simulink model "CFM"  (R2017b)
settings: Solver=FixedStepDiscrete  StartTime=0.0  StopTime=10.0  FixedStep=0.01  RelTol=1e-3  EnableMultiTasking=on
undefined symbols (not defined in the file): ASWTYPE_FALSE, CaCFM_BusBarCell_enum, CaCFM_NTCTemp_enum, CcCFM_AFEAdcRelatedErrDeb_ms, CcCFM_AFECellTempUpdErrDeb_ms, CcCFM_AFECellVoltLineOpenDeb_ms, CcCFM_AFECellVoltUpdErrDeb_ms, CcCFM_AFEComLostDeb_ms, CcCFM_AFEDiagModeExitErrDeb_ms, CcCFM_AFEGpioLineOpenDeb_ms, CcCFM_AFEOtherErrDeb_ms, CcCFM_AFESampleErrDeb_ms, CFM_CONST0_NUMB, CFM_CONST14_NUMB, CFM_CONST1_NUMB, CFM_CONST6_NUMB, CFM_CONST8_NUMB, CFM_RUNTIME20_MS, Enum_CFMBusBarCell, Enum_CFMNTCTemp
libraries: AIWAYS_Powertrain_BMS_lib x22

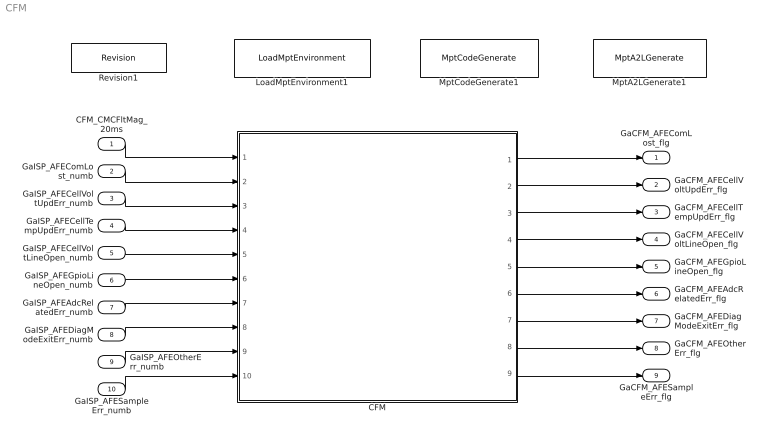
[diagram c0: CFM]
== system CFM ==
  CFM_CMCFltMag_20ms : Inport
  GaISP_AFEComLost_numb : Inport  Port=2
  GaISP_AFECellVoltUpdErr_numb : Inport  Port=3
  GaISP_AFECellTempUpdErr_numb : Inport  Port=4
  GaISP_AFECellVoltLineOpen_numb : Inport  Port=5
  GaISP_AFEGpioLineOpen_numb : Inport  Port=6
  GaISP_AFEAdcRelatedErr_numb : Inport  Port=7
  GaISP_AFEDiagModeExitErr_numb : Inport  Port=8
  GaISP_AFEOtherErr_numb : Inport  Port=9
  GaISP_AFESampleErr_numb : Inport  Port=10
  CFM : Subsystem
  LoadMptEnvironment1 : AIWAYS_Powertrain_BMS_lib/Config/LoadMptEnvironment  ProjectName=861B  SuppierID=NewPlatformUAES
  MptA2LGenerate1 : AIWAYS_Powertrain_BMS_lib/Config/MptA2LGenerate  SystemSampleTime=-1
  MptCodeGenerate1 : AIWAYS_Powertrain_BMS_lib/Config/MptCodeGenerate  SystemSampleTime=-1
  Revision1 : AIWAYS_Powertrain_BMS_lib/Config/Revision  curVersion='M100C100'  newVersion='M100C100'
  GaCFM_AFEComLost_flg : Outport
  GaCFM_AFECellVoltUpdErr_flg : Outport  Port=2
  GaCFM_AFECellTempUpdErr_flg : Outport  Port=3
  GaCFM_AFECellVoltLineOpen_flg : Outport  Port=4
  GaCFM_AFEGpioLineOpen_flg : Outport  Port=5
  GaCFM_AFEAdcRelatedErr_flg : Outport  Port=6
  GaCFM_AFEDiagModeExitErr_flg : Outport  Port=7
  GaCFM_AFEOtherErr_flg : Outport  Port=8
  GaCFM_AFESampleErr_flg : Outport  Port=9
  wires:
  GaISP_AFEComLost_numb/1 -> CFM/2(GaISP_AFEComLost_numb)
  GaISP_AFECellVoltUpdErr_numb/1 -> CFM/3(GaISP_AFECellVoltUpdErr_numb)
  GaISP_AFECellTempUpdErr_numb/1 -> CFM/4(GaISP_AFECellTempUpdErr_numb)
  GaISP_AFECellVoltLineOpen_numb/1 -> CFM/5(GaISP_AFECellVoltLineOpen_numb)
  GaISP_AFEGpioLineOpen_numb/1 -> CFM/6(GaISP_AFEGpioLineOpen_numb)
  GaISP_AFEAdcRelatedErr_numb/1 -> CFM/7(GaISP_AFEAdcRelatedErr_numb)
  GaISP_AFEDiagModeExitErr_numb/1 -> CFM/8(GaISP_AFEDiagModeExitErr_numb)
  GaISP_AFEOtherErr_numb/1 -> CFM/9(GaISP_AFEOtherErr_numb)
  GaISP_AFESampleErr_numb/1 -> CFM/10(GaISP_AFESampleErr_numb)
  CFM_CMCFltMag_20ms/1 -> CFM/1(CFM_CMCFltMag_20ms)
  CFM/1(GaCFM_AFEComLost_flg) -> GaCFM_AFEComLost_flg/1
  CFM/2(GaCFM_AFECellVoltUpdErr_flg) -> GaCFM_AFECellVoltUpdErr_flg/1
  CFM/3(GaCFM_AFECellTempUpdErr_flg) -> GaCFM_AFECellTempUpdErr_flg/1
  CFM/4(GaCFM_AFECellVoltLineOpen_flg) -> GaCFM_AFECellVoltLineOpen_flg/1
  CFM/5(GaCFM_AFEGpioLineOpen_flg) -> GaCFM_AFEGpioLineOpen_flg/1
  CFM/6(GaCFM_AFEAdcRelatedErr_flg) -> GaCFM_AFEAdcRelatedErr_flg/1
  CFM/7(GaCFM_AFEDiagModeExitErr_flg) -> GaCFM_AFEDiagModeExitErr_flg/1
  CFM/8(GaCFM_AFEOtherErr_flg) -> GaCFM_AFEOtherErr_flg/1
  CFM/9(GaCFM_AFESampleErr_flg) -> GaCFM_AFESampleErr_flg/1

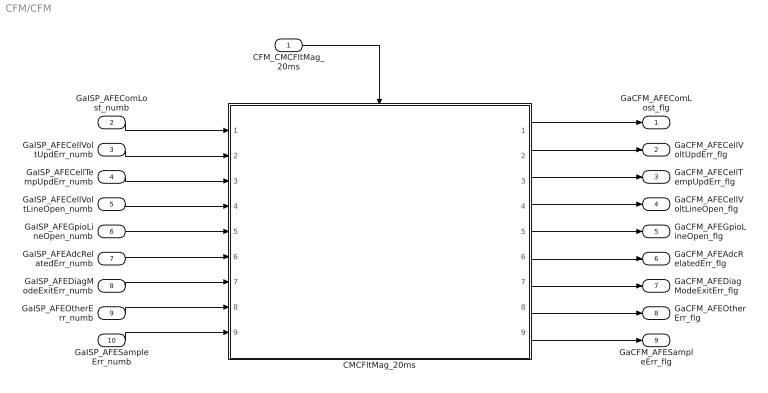
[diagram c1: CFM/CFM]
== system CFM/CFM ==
  CFM_CMCFltMag_20ms : Inport
  GaISP_AFEComLost_numb : Inport  Port=2
  GaISP_AFECellVoltUpdErr_numb : Inport  Port=3
  GaISP_AFECellTempUpdErr_numb : Inport  Port=4
  GaISP_AFECellVoltLineOpen_numb : Inport  Port=5
  GaISP_AFEGpioLineOpen_numb : Inport  Port=6
  GaISP_AFEAdcRelatedErr_numb : Inport  Port=7
  GaISP_AFEDiagModeExitErr_numb : Inport  Port=8
  GaISP_AFEOtherErr_numb : Inport  Port=9
  GaISP_AFESampleErr_numb : Inport  Port=10
  CMCFltMag_20ms : Subsystem
  GaCFM_AFEComLost_flg : Outport
  GaCFM_AFECellVoltUpdErr_flg : Outport  Port=2
  GaCFM_AFECellTempUpdErr_flg : Outport  Port=3
  GaCFM_AFECellVoltLineOpen_flg : Outport  Port=4
  GaCFM_AFEGpioLineOpen_flg : Outport  Port=5
  GaCFM_AFEAdcRelatedErr_flg : Outport  Port=6
  GaCFM_AFEDiagModeExitErr_flg : Outport  Port=7
  GaCFM_AFEOtherErr_flg : Outport  Port=8
  GaCFM_AFESampleErr_flg : Outport  Port=9
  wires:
  CFM_CMCFltMag_20ms/1 -> CMCFltMag_20ms/Trigger
  GaISP_AFEComLost_numb/1 -> CMCFltMag_20ms/1(GaISP_AFEComLost_numb)
  GaISP_AFECellVoltUpdErr_numb/1 -> CMCFltMag_20ms/2(GaISP_AFECellVoltUpdErr_numb)
  GaISP_AFECellTempUpdErr_numb/1 -> CMCFltMag_20ms/3(GaISP_AFECellTempUpdErr_numb)
  GaISP_AFECellVoltLineOpen_numb/1 -> CMCFltMag_20ms/4(GaISP_AFECellVoltLineOpen_numb)
  GaISP_AFEGpioLineOpen_numb/1 -> CMCFltMag_20ms/5(GaISP_AFEGpioLineOpen_numb)
  GaISP_AFEAdcRelatedErr_numb/1 -> CMCFltMag_20ms/6(GaISP_AFEAdcRelatedErr_numb)
  GaISP_AFEDiagModeExitErr_numb/1 -> CMCFltMag_20ms/7(GaISP_AFEDiagModeExitErr_numb)
  GaISP_AFEOtherErr_numb/1 -> CMCFltMag_20ms/8(GaISP_AFEOtherErr_numb)
  GaISP_AFESampleErr_numb/1 -> CMCFltMag_20ms/9(GaISP_AFESampleErr_numb)
  CMCFltMag_20ms/1(GaCFM_AFEComLost_flg) -> GaCFM_AFEComLost_flg/1
  CMCFltMag_20ms/2(GaCFM_AFECellVoltUpdErr_flg) -> GaCFM_AFECellVoltUpdErr_flg/1
  CMCFltMag_20ms/3(GaCFM_AFECellTempUpdErr_flg) -> GaCFM_AFECellTempUpdErr_flg/1
  CMCFltMag_20ms/4(GaCFM_AFECellVoltLineOpen_flg) -> GaCFM_AFECellVoltLineOpen_flg/1
  CMCFltMag_20ms/5(GaCFM_AFEGpioLineOpen_flg) -> GaCFM_AFEGpioLineOpen_flg/1
  CMCFltMag_20ms/6(GaCFM_AFEAdcRelatedErr_flg) -> GaCFM_AFEAdcRelatedErr_flg/1
  CMCFltMag_20ms/7(GaCFM_AFEDiagModeExitErr_flg) -> GaCFM_AFEDiagModeExitErr_flg/1
  CMCFltMag_20ms/8(GaCFM_AFEOtherErr_flg) -> GaCFM_AFEOtherErr_flg/1
  CMCFltMag_20ms/9(GaCFM_AFESampleErr_flg) -> GaCFM_AFESampleErr_flg/1

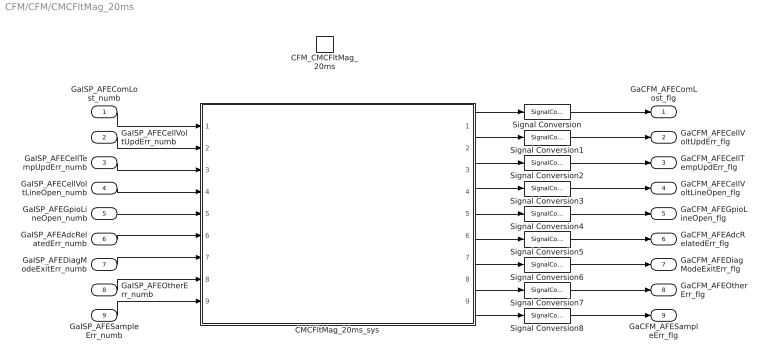
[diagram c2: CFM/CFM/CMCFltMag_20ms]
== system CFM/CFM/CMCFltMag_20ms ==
  GaISP_AFEComLost_numb : Inport
  GaISP_AFECellVoltUpdErr_numb : Inport  Port=2
  GaISP_AFECellTempUpdErr_numb : Inport  Port=3
  GaISP_AFECellVoltLineOpen_numb : Inport  Port=4
  GaISP_AFEGpioLineOpen_numb : Inport  Port=5
  GaISP_AFEAdcRelatedErr_numb : Inport  Port=6
  GaISP_AFEDiagModeExitErr_numb : Inport  Port=7
  GaISP_AFEOtherErr_numb : Inport  Port=8
  GaISP_AFESampleErr_numb : Inport  Port=9
  CFM_CMCFltMag_20ms : TriggerPort  TriggerType=function-call  VariantControl=(inherit)
  CMCFltMag_20ms_sys : Subsystem
  Signal Conversion{,1..8} (9 alike) : SignalConversion  ConversionOutput=Contiguous copy  OverrideOpt=off
  GaCFM_AFEComLost_flg : Outport
  GaCFM_AFECellVoltUpdErr_flg : Outport  Port=2
  GaCFM_AFECellTempUpdErr_flg : Outport  Port=3
  GaCFM_AFECellVoltLineOpen_flg : Outport  Port=4
  GaCFM_AFEGpioLineOpen_flg : Outport  Port=5
  GaCFM_AFEAdcRelatedErr_flg : Outport  Port=6
  GaCFM_AFEDiagModeExitErr_flg : Outport  Port=7
  GaCFM_AFEOtherErr_flg : Outport  Port=8
  GaCFM_AFESampleErr_flg : Outport  Port=9
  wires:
  GaISP_AFEComLost_numb/1 -> CMCFltMag_20ms_sys/1(GaISP_AFEComLost_numb)
  GaISP_AFECellVoltUpdErr_numb/1 -> CMCFltMag_20ms_sys/2(GaISP_AFECellVoltUpdErr_numb)
  GaISP_AFECellTempUpdErr_numb/1 -> CMCFltMag_20ms_sys/3(GaISP_AFECellTempUpdErr_numb)
  GaISP_AFECellVoltLineOpen_numb/1 -> CMCFltMag_20ms_sys/4(GaISP_AFECellVoltLineOpen_numb)
  GaISP_AFEGpioLineOpen_numb/1 -> CMCFltMag_20ms_sys/5(GaISP_AFEGpioLineOpen_numb)
  GaISP_AFEAdcRelatedErr_numb/1 -> CMCFltMag_20ms_sys/6(GaISP_AFEAdcRelatedErr_numb)
  GaISP_AFEDiagModeExitErr_numb/1 -> CMCFltMag_20ms_sys/7(GaISP_AFEDiagModeExitErr_numb)
  GaISP_AFEOtherErr_numb/1 -> CMCFltMag_20ms_sys/8(GaISP_AFEOtherErr_numb)
  GaISP_AFESampleErr_numb/1 -> CMCFltMag_20ms_sys/9(GaISP_AFESampleErr_numb)
  CMCFltMag_20ms_sys/1(GaCFM_AFEComLost_flg) -> Signal Conversion/1
  CMCFltMag_20ms_sys/2(GaCFM_AFECellVoltUpdErr_flg) -> Signal Conversion1/1
  CMCFltMag_20ms_sys/3(GaCFM_AFECellTempUpdErr_flg) -> Signal Conversion2/1
  CMCFltMag_20ms_sys/4(GaCFM_AFECellVoltLineOpen_flg) -> Signal Conversion3/1
  CMCFltMag_20ms_sys/5(GaCFM_AFEGpioLineOpen_flg) -> Signal Conversion4/1
  CMCFltMag_20ms_sys/6(GaCFM_AFEAdcRelatedErr_flg) -> Signal Conversion5/1
  CMCFltMag_20ms_sys/7(GaCFM_AFEDiagModeExitErr_flg) -> Signal Conversion6/1
  CMCFltMag_20ms_sys/8(GaCFM_AFEOtherErr_flg) -> Signal Conversion7/1
  CMCFltMag_20ms_sys/9(GaCFM_AFESampleErr_flg) -> Signal Conversion8/1
  Signal Conversion/1 -> GaCFM_AFEComLost_flg/1
  Signal Conversion1/1 -> GaCFM_AFECellVoltUpdErr_flg/1
  Signal Conversion2/1 -> GaCFM_AFECellTempUpdErr_flg/1
  Signal Conversion3/1 -> GaCFM_AFECellVoltLineOpen_flg/1
  Signal Conversion4/1 -> GaCFM_AFEGpioLineOpen_flg/1
  Signal Conversion5/1 -> GaCFM_AFEAdcRelatedErr_flg/1
  Signal Conversion6/1 -> GaCFM_AFEDiagModeExitErr_flg/1
  Signal Conversion7/1 -> GaCFM_AFEOtherErr_flg/1
  Signal Conversion8/1 -> GaCFM_AFESampleErr_flg/1

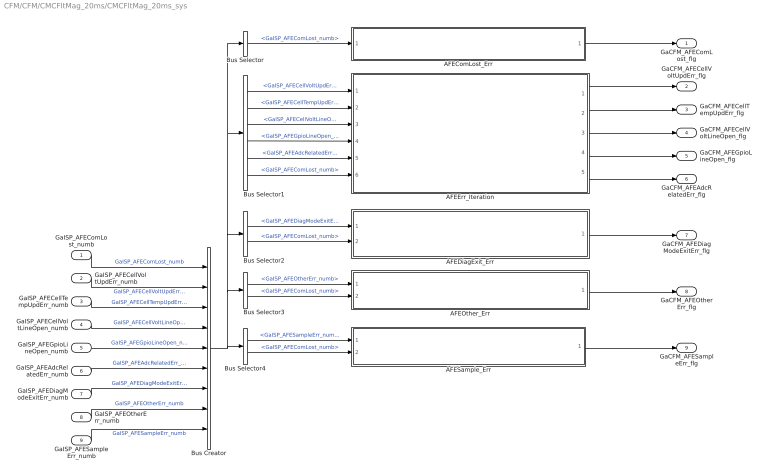
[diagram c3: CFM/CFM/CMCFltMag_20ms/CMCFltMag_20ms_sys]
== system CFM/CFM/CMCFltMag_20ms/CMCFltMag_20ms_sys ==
  GaISP_AFEComLost_numb : Inport
  GaISP_AFECellVoltUpdErr_numb : Inport  Port=2
  GaISP_AFECellTempUpdErr_numb : Inport  Port=3
  GaISP_AFECellVoltLineOpen_numb : Inport  Port=4
  GaISP_AFEGpioLineOpen_numb : Inport  Port=5
  GaISP_AFEAdcRelatedErr_numb : Inport  Port=6
  GaISP_AFEDiagModeExitErr_numb : Inport  Port=7
  GaISP_AFEOtherErr_numb : Inport  Port=8
  GaISP_AFESampleErr_numb : Inport  Port=9
  AFEComLost_Err : Subsystem
  AFEDiagExit_Err : Subsystem
  AFEErr_Iteration : Subsystem
  AFEOther_Err : Subsystem
  AFESample_Err : Subsystem
  Bus Creator : BusCreator  Inputs=9
  Bus Selector : BusSelector  OutputSignals=GaISP_AFEComLost_numb
  Bus Selector1 : BusSelector  OutputSignals=GaISP_AFECellVoltUpdErr_numb,GaISP_AFECellTempUpdErr_numb,GaISP_AFECellVoltLineOpen_numb,GaISP_AFEGpioLineOpen_numb,GaISP_AFEAdcRelatedErr_numb,GaISP_AFEComLost_numb
  Bus Selector2 : BusSelector  OutputSignals=GaISP_AFEDiagModeExitErr_numb,GaISP_AFEComLost_numb
  Bus Selector3 : BusSelector  OutputSignals=GaISP_AFEOtherErr_numb,GaISP_AFEComLost_numb
  Bus Selector4 : BusSelector  OutputSignals=GaISP_AFESampleErr_numb,GaISP_AFEComLost_numb
  GaCFM_AFEComLost_flg : Outport
  GaCFM_AFECellVoltUpdErr_flg : Outport  Port=2
  GaCFM_AFECellTempUpdErr_flg : Outport  Port=3
  GaCFM_AFECellVoltLineOpen_flg : Outport  Port=4
  GaCFM_AFEGpioLineOpen_flg : Outport  Port=5
  GaCFM_AFEAdcRelatedErr_flg : Outport  Port=6
  GaCFM_AFEDiagModeExitErr_flg : Outport  Port=7
  GaCFM_AFEOtherErr_flg : Outport  Port=8
  GaCFM_AFESampleErr_flg : Outport  Port=9
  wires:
  AFEComLost_Err/1(GaCFM_AFEComLost_flg) -> GaCFM_AFEComLost_flg/1
  AFEDiagExit_Err/1(GaCFM_AFEDiagModeExitErr_flg) -> GaCFM_AFEDiagModeExitErr_flg/1
  AFEOther_Err/1(GaCFM_AFEOtherErr_flg) -> GaCFM_AFEOtherErr_flg/1
  AFESample_Err/1(GaCFM_AFESampleErr_flg) -> GaCFM_AFESampleErr_flg/1
  AFEErr_Iteration/1(GaCFM_AFECellVoltUpdErr_flg) -> GaCFM_AFECellVoltUpdErr_flg/1
  AFEErr_Iteration/2(GaCFM_AFECellTempUpdErr_flg) -> GaCFM_AFECellTempUpdErr_flg/1
  AFEErr_Iteration/3(GaCFM_AFECellVoltLineOpen_flg) -> GaCFM_AFECellVoltLineOpen_flg/1
  AFEErr_Iteration/4(GaCFM_AFEGpioLineOpen_flg) -> GaCFM_AFEGpioLineOpen_flg/1
  AFEErr_Iteration/5(GaCFM_AFEAdcRelatedErr_flg) -> GaCFM_AFEAdcRelatedErr_flg/1
  GaISP_AFEComLost_numb/1 -> Bus Creator/1  "GaISP_AFEComLost_numb"
  GaISP_AFECellVoltUpdErr_numb/1 -> Bus Creator/2  "GaISP_AFECellVoltUpdErr_numb"
  GaISP_AFECellTempUpdErr_numb/1 -> Bus Creator/3  "GaISP_AFECellTempUpdErr_numb"
  GaISP_AFECellVoltLineOpen_numb/1 -> Bus Creator/4  "GaISP_AFECellVoltLineOpen_numb"
  GaISP_AFEGpioLineOpen_numb/1 -> Bus Creator/5  "GaISP_AFEGpioLineOpen_numb"
  GaISP_AFEAdcRelatedErr_numb/1 -> Bus Creator/6  "GaISP_AFEAdcRelatedErr_numb"
  GaISP_AFEDiagModeExitErr_numb/1 -> Bus Creator/7  "GaISP_AFEDiagModeExitErr_numb"
  GaISP_AFEOtherErr_numb/1 -> Bus Creator/8  "GaISP_AFEOtherErr_numb"
  GaISP_AFESampleErr_numb/1 -> Bus Creator/9  "GaISP_AFESampleErr_numb"
  Bus Creator/1 -> Bus Selector/1, Bus Selector1/1, Bus Selector2/1, Bus Selector3/1, Bus Selector4/1
  Bus Selector/1 -> AFEComLost_Err/1(GaISP_AFEComLost_numb)  "<GaISP_AFEComLost_numb>"
  Bus Selector1/1 -> AFEErr_Iteration/1(GaISP_AFECellVoltUpdErr_numb)  "<GaISP_AFECellVoltUpdErr_numb>"
  Bus Selector1/2 -> AFEErr_Iteration/2(GaISP_AFECellTempUpdErr_numb)  "<GaISP_AFECellTempUpdErr_numb>"
  Bus Selector1/3 -> AFEErr_Iteration/3(GaISP_AFECellVoltLineOpen_numb)  "<GaISP_AFECellVoltLineOpen_numb>"
  Bus Selector1/4 -> AFEErr_Iteration/4(GaISP_AFEGpioLineOpen_numb)  "<GaISP_AFEGpioLineOpen_numb>"
  Bus Selector1/5 -> AFEErr_Iteration/5(GaISP_AFEAdcRelatedErr_numb)  "<GaISP_AFEAdcRelatedErr_numb>"
  Bus Selector1/6 -> AFEErr_Iteration/6(GaISP_AFEComLost_numb)  "<GaISP_AFEComLost_numb>"
  Bus Selector2/1 -> AFEDiagExit_Err/1(GaISP_AFEDiagModeExitErr_numb)  "<GaISP_AFEDiagModeExitErr_numb>"
  Bus Selector2/2 -> AFEDiagExit_Err/2(GaISP_AFEComLost_numb)  "<GaISP_AFEComLost_numb>"
  Bus Selector3/1 -> AFEOther_Err/1(GaISP_AFEOtherErr_numb)  "<GaISP_AFEOtherErr_numb>"
  Bus Selector3/2 -> AFEOther_Err/2(GaISP_AFEComLost_numb)  "<GaISP_AFEComLost_numb>"
  Bus Selector4/2 -> AFESample_Err/2(GaISP_AFEComLost_numb)  "<GaISP_AFEComLost_numb>"
  Bus Selector4/1 -> AFESample_Err/1(GaISP_AFESampleErr_numb)  "<GaISP_AFESampleErr_numb>"

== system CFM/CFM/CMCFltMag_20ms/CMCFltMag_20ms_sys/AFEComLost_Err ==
  GaISP_AFEComLost_numb : Inport
  BMSDelay : AIWAYS_Powertrain_BMS_lib/Debounce & Delay/BMSDelay
  CFM_GaCFM_AFEComLost_flg : AIWAYS_Powertrain_BMS_lib/Signals/OverWrite  OverWrite_Value=CaCFM_AFEComLostOvr_flg  OverWrite_flag=CbCFM_AFEComLostOvrSwt_flg
  Constant1 : Constant  Value=CFM_RUNTIME20_MS
  Constant3 : Constant  Value=CFM_CONST0_NUMB
  Constant5 : Constant  Value=CcCFM_AFEComLostDeb_ms
  Relational Operator2 : RelationalOperator  Operator=~=  OutDataTypeStr=boolean
  GaCFM_AFEComLost_flg : Outport
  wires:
  GaISP_AFEComLost_numb/1 -> Relational Operator2/1
  Constant3/1 -> Relational Operator2/2
  CFM_GaCFM_AFEComLost_flg/1 -> GaCFM_AFEComLost_flg/1  "GaCFM_AFEComLost_flg"
  Relational Operator2/1 -> BMSDelay/1  "LaCFM_AFEComLost_flg"
  BMSDelay/1 -> CFM_GaCFM_AFEComLost_flg/1
  Constant1/1 -> BMSDelay/2
  Constant5/1 -> BMSDelay/3

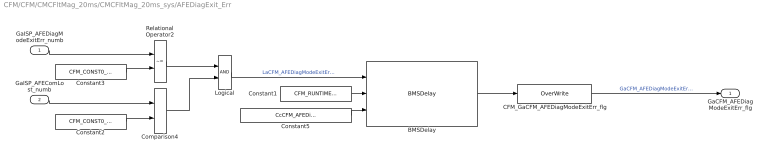
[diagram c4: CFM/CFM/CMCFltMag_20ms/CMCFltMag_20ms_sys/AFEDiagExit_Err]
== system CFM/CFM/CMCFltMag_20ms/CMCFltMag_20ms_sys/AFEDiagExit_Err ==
  GaISP_AFEDiagModeExitErr_numb : Inport
  GaISP_AFEComLost_numb : Inport  Port=2
  BMSDelay : AIWAYS_Powertrain_BMS_lib/Debounce & Delay/BMSDelay
  CFM_GaCFM_AFEDiagModeExitErr_flg : AIWAYS_Powertrain_BMS_lib/Signals/OverWrite  OverWrite_Value=CaCFM_AFEDiagModeExitErrOvr_flg  OverWrite_flag=CbCFM_AFEDiagModeExitErrOvrSwt_flg
  Comparison4 : RelationalOperator  Operator===  OutDataTypeStr=boolean
  Constant1 : Constant  Value=CFM_RUNTIME20_MS
  Constant2 : Constant  Value=CFM_CONST0_NUMB
  Constant3 : Constant  Value=CFM_CONST0_NUMB
  Constant5 : Constant  Value=CcCFM_AFEDiagModeExitErrDeb_ms
  Logical : Logic  OutDataTypeStr=boolean
  Relational Operator2 : RelationalOperator  Operator=~=  OutDataTypeStr=boolean
  GaCFM_AFEDiagModeExitErr_flg : Outport
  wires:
  Constant3/1 -> Relational Operator2/2
  GaISP_AFEDiagModeExitErr_numb/1 -> Relational Operator2/1
  CFM_GaCFM_AFEDiagModeExitErr_flg/1 -> GaCFM_AFEDiagModeExitErr_flg/1  "GaCFM_AFEDiagModeExitErr_flg"
  Constant5/1 -> BMSDelay/3
  Constant1/1 -> BMSDelay/2
  BMSDelay/1 -> CFM_GaCFM_AFEDiagModeExitErr_flg/1
  Constant2/1 -> Comparison4/2
  GaISP_AFEComLost_numb/1 -> Comparison4/1
  Relational Operator2/1 -> Logical/1
  Comparison4/1 -> Logical/2
  Logical/1 -> BMSDelay/1  "LaCFM_AFEDiagModeExitErr_flg"

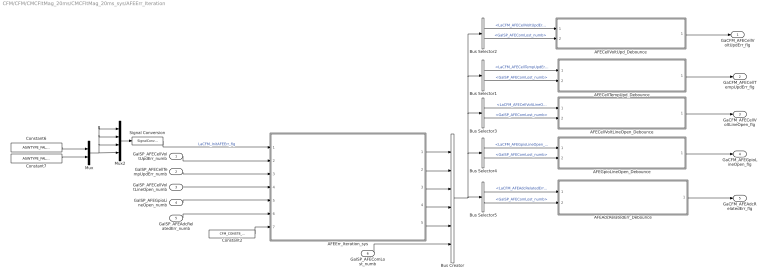
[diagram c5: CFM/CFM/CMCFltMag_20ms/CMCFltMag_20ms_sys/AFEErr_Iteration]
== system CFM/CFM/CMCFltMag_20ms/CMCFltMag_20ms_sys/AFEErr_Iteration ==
  GaISP_AFECellVoltUpdErr_numb : Inport
  GaISP_AFECellTempUpdErr_numb : Inport  Port=2
  GaISP_AFECellVoltLineOpen_numb : Inport  Port=3
  GaISP_AFEGpioLineOpen_numb : Inport  Port=4
  GaISP_AFEAdcRelatedErr_numb : Inport  Port=5
  GaISP_AFEComLost_numb : Inport  Port=6
  AFEAdcRelatedErr_Debounce : Subsystem
  AFECellTempUpd_Debounce : Subsystem
  AFECellVoltLineOpen_Debounce : Subsystem
  AFECellVoltUpd_Debounce : Subsystem
  AFEErr_Iteration_sys : Subsystem
  AFEGpioLineOpen_Debounce : Subsystem
  Bus Creator : BusCreator  Inputs=6
  Bus Selector1 : BusSelector  OutputSignals=LaCFM_AFECellTempUpdErr_flg,GaISP_AFEComLost_numb
  Bus Selector2 : BusSelector  OutputSignals=LaCFM_AFECellVoltUpdErr_flg,GaISP_AFEComLost_numb
  Bus Selector3 : BusSelector  OutputSignals=LaCFM_AFECellVoltLineOpen_flg,GaISP_AFEComLost_numb
  Bus Selector4 : BusSelector  OutputSignals=LaCFM_AFEGpioLineOpen_flg,GaISP_AFEComLost_numb
  Bus Selector5 : BusSelector  OutputSignals=LaCFM_AFEAdcRelatedErr_flg,GaISP_AFEComLost_numb
  Constant2 : Constant  Value=CFM_CONST8_NUMB
  Constant6 : Constant  Value=ASWTYPE_FALSE
  Constant7 : Constant  Value=ASWTYPE_FALSE
  Mux : Mux  Inputs=2
  Mux2 : Mux
  Signal Conversion : SignalConversion  ConversionOutput=Contiguous copy  OverrideOpt=off
  GaCFM_AFECellVoltUpdErr_flg : Outport
  GaCFM_AFECellTempUpdErr_flg : Outport  Port=2
  GaCFM_AFECellVoltLineOpen_flg : Outport  Port=3
  GaCFM_AFEGpioLineOpen_flg : Outport  Port=4
  GaCFM_AFEAdcRelatedErr_flg : Outport  Port=5
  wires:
  GaISP_AFEGpioLineOpen_numb/1 -> AFEErr_Iteration_sys/5(GaISP_AFEGpioLineOpen_numb)
  GaISP_AFECellTempUpdErr_numb/1 -> AFEErr_Iteration_sys/3(GaISP_AFECellTempUpdErr_numb)
  Signal Conversion/1 -> AFEErr_Iteration_sys/1(LaCFM_InitAFEErr_flg)  "LaCFM_InitAFEErr_flg"
  GaISP_AFECellVoltLineOpen_numb/1 -> AFEErr_Iteration_sys/4(GaISP_AFECellVoltLineOpen_numb)
  Constant2/1 -> AFEErr_Iteration_sys/7(CFM_CONST8_NUMB)
  GaISP_AFECellVoltUpdErr_numb/1 -> AFEErr_Iteration_sys/2(GaISP_AFECellVoltUpdErr_numb)
  GaISP_AFEAdcRelatedErr_numb/1 -> AFEErr_Iteration_sys/6(GaISP_AFEAdcRelatedErr_numb)
  Constant6/1 -> Mux/1
  Mux2/1 -> Signal Conversion/1
  Mux/1 -> Mux2/1, Mux2/2, Mux2/3, Mux2/4
  Constant7/1 -> Mux/2
  AFECellVoltUpd_Debounce/1(GaCFM_AFECellVoltUpdErr_flg) -> GaCFM_AFECellVoltUpdErr_flg/1
  AFECellTempUpd_Debounce/1(GaCFM_AFECellTempUpdErr_flg) -> GaCFM_AFECellTempUpdErr_flg/1
  AFECellVoltLineOpen_Debounce/1(GaCFM_AFECellVoltLineOpen_flg) -> GaCFM_AFECellVoltLineOpen_flg/1
  AFEGpioLineOpen_Debounce/1(GaCFM_AFEGpioLineOpen_flg) -> GaCFM_AFEGpioLineOpen_flg/1
  AFEAdcRelatedErr_Debounce/1(GaCFM_AFEAdcRelatedErr_flg) -> GaCFM_AFEAdcRelatedErr_flg/1
  AFEErr_Iteration_sys/1(LaCFM_AFECellVoltUpdErr_flg) -> Bus Creator/1
  AFEErr_Iteration_sys/2(LaCFM_AFECellTempUpdErr_flg) -> Bus Creator/2
  AFEErr_Iteration_sys/3(LaCFM_AFECellVoltLineOpen_flg) -> Bus Creator/3
  AFEErr_Iteration_sys/4(LaCFM_AFEGpioLineOpen_flg) -> Bus Creator/4
  AFEErr_Iteration_sys/5(LaCFM_AFEAdcRelatedErr_flg) -> Bus Creator/5
  GaISP_AFEComLost_numb/1 -> Bus Creator/6
  Bus Creator/1 -> Bus Selector1/1, Bus Selector2/1, Bus Selector3/1, Bus Selector4/1, Bus Selector5/1
  Bus Selector2/1 -> AFECellVoltUpd_Debounce/1(LaCFM_AFECellVoltUpdErr_flg)  "<LaCFM_AFECellVoltUpdErr_flg>"
  Bus Selector2/2 -> AFECellVoltUpd_Debounce/2(GaISP_AFEComLost_numb)  "<GaISP_AFEComLost_numb>"
  Bus Selector1/1 -> AFECellTempUpd_Debounce/1(LaCFM_AFECellTempUpdErr_flg)  "<LaCFM_AFECellTempUpdErr_flg>"
  Bus Selector1/2 -> AFECellTempUpd_Debounce/2(GaISP_AFEComLost_numb)  "<GaISP_AFEComLost_numb>"
  Bus Selector3/1 -> AFECellVoltLineOpen_Debounce/1(LaCFM_AFECellVoltLineOpen_flg)  "<LaCFM_AFECellVoltLineOpen_flg>"
  Bus Selector3/2 -> AFECellVoltLineOpen_Debounce/2(GaISP_AFEComLost_numb)  "<GaISP_AFEComLost_numb>"
  Bus Selector4/1 -> AFEGpioLineOpen_Debounce/1(LaCFM_AFEGpioLineOpen_flg)  "<LaCFM_AFEGpioLineOpen_flg>"
  Bus Selector4/2 -> AFEGpioLineOpen_Debounce/2(GaISP_AFEComLost_numb)  "<GaISP_AFEComLost_numb>"
  Bus Selector5/1 -> AFEAdcRelatedErr_Debounce/1(LaCFM_AFEAdcRelatedErr_flg)  "<LaCFM_AFEAdcRelatedErr_flg>"
  Bus Selector5/2 -> AFEAdcRelatedErr_Debounce/2(GaISP_AFEComLost_numb)  "<GaISP_AFEComLost_numb>"

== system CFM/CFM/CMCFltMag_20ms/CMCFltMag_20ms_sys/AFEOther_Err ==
  GaISP_AFEOtherErr_numb : Inport
  GaISP_AFEComLost_numb : Inport  Port=2
  BMSDelay : AIWAYS_Powertrain_BMS_lib/Debounce & Delay/BMSDelay
  CFM_GaCFM_AFEOtherErr_flg : AIWAYS_Powertrain_BMS_lib/Signals/OverWrite  OverWrite_Value=CaCFM_AFEOtherErrOvr_flg  OverWrite_flag=CbCFM_AFEOtherErrOvrSwt_flg
  Comparison4 : RelationalOperator  Operator===  OutDataTypeStr=boolean
  Constant1 : Constant  Value=CFM_RUNTIME20_MS
  Constant3 : Constant  Value=CFM_CONST0_NUMB
  Constant5 : Constant  Value=CcCFM_AFEOtherErrDeb_ms
  Constant6 : Constant  Value=CFM_CONST0_NUMB
  Logical : Logic  OutDataTypeStr=boolean
  Relational Operator2 : RelationalOperator  Operator=~=  OutDataTypeStr=boolean
  GaCFM_AFEOtherErr_flg : Outport
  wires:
  GaISP_AFEOtherErr_numb/1 -> Relational Operator2/1
  Constant3/1 -> Relational Operator2/2
  CFM_GaCFM_AFEOtherErr_flg/1 -> GaCFM_AFEOtherErr_flg/1  "GaCFM_AFEOtherErr_flg"
  Constant5/1 -> BMSDelay/3
  Constant1/1 -> BMSDelay/2
  BMSDelay/1 -> CFM_GaCFM_AFEOtherErr_flg/1
  Relational Operator2/1 -> Logical/1
  Constant6/1 -> Comparison4/2
  GaISP_AFEComLost_numb/1 -> Comparison4/1
  Comparison4/1 -> Logical/2
  Logical/1 -> BMSDelay/1  "LaCFM_AFEOtherErr_flg"

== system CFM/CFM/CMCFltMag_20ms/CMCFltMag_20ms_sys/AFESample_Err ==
  GaISP_AFESampleErr_numb : Inport
  GaISP_AFEComLost_numb : Inport  Port=2
  BMSDelay : AIWAYS_Powertrain_BMS_lib/Debounce & Delay/BMSDelay
  CFM_GaCFM_AFESampleErr_flg : AIWAYS_Powertrain_BMS_lib/Signals/OverWrite  OverWrite_Value=CaCFM_AFESampleErrOvr_flg  OverWrite_flag=CbCFM_AFESampleErrOvrSwt_flg
  Constant1 : Constant  Value=CFM_RUNTIME20_MS
  Constant2 : Constant  Value=CFM_CONST0_NUMB
  Constant3 : Constant  Value=CFM_CONST0_NUMB
  Constant5 : Constant  Value=CcCFM_AFESampleErrDeb_ms
  Logical : Logic  OutDataTypeStr=boolean
  Relational Operator1 : RelationalOperator  Operator===  OutDataTypeStr=boolean
  Relational Operator2 : RelationalOperator  Operator=~=  OutDataTypeStr=boolean
  GaCFM_AFESampleErr_flg : Outport
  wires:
  GaISP_AFESampleErr_numb/1 -> Relational Operator2/1
  Constant3/1 -> Relational Operator2/2
  CFM_GaCFM_AFESampleErr_flg/1 -> GaCFM_AFESampleErr_flg/1  "GaCFM_AFESampleErr_flg"
  Constant5/1 -> BMSDelay/3
  Constant1/1 -> BMSDelay/2
  BMSDelay/1 -> CFM_GaCFM_AFESampleErr_flg/1
  Logical/1 -> BMSDelay/1  "LaCFM_AFESampleErr_flg"
  Constant2/1 -> Relational Operator1/2
  GaISP_AFEComLost_numb/1 -> Relational Operator1/1
  Relational Operator2/1 -> Logical/1
  Relational Operator1/1 -> Logical/2

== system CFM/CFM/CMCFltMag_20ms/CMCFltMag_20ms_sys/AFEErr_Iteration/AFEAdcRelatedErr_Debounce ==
  LaCFM_AFEAdcRelatedErr_flg : Inport
  GaISP_AFEComLost_numb : Inport  Port=2
  BMSDelay : AIWAYS_Powertrain_BMS_lib/Debounce & Delay/BMSDelay
  CFM_GaCFM_AFEAdcRelatedErr_flg : AIWAYS_Powertrain_BMS_lib/Signals/OverWrite  OverWrite_Value=CaCFM_AFEAdcRelatedErrOvr_flg  OverWrite_flag=CbCFM_AFEAdcRelatedErrOvrSwt_flg
  Comparison4 : RelationalOperator  Operator===  OutDataTypeStr=boolean
  Constant1 : Constant  Value=CFM_RUNTIME20_MS
  Constant3 : Constant  Value=CFM_CONST0_NUMB
  Constant5 : Constant  Value=CcCFM_AFEAdcRelatedErrDeb_ms
  Logical : Logic  OutDataTypeStr=boolean
  GaCFM_AFEAdcRelatedErr_flg : Outport
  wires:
  LaCFM_AFEAdcRelatedErr_flg/1 -> Logical/1
  CFM_GaCFM_AFEAdcRelatedErr_flg/1 -> GaCFM_AFEAdcRelatedErr_flg/1  "GaCFM_AFEAdcRelatedErr_flg"
  BMSDelay/1 -> CFM_GaCFM_AFEAdcRelatedErr_flg/1
  Constant1/1 -> BMSDelay/2
  Constant5/1 -> BMSDelay/3
  GaISP_AFEComLost_numb/1 -> Comparison4/1
  Comparison4/1 -> Logical/2
  Logical/1 -> BMSDelay/1
  Constant3/1 -> Comparison4/2

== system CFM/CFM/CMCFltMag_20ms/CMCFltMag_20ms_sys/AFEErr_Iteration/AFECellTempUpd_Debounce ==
  LaCFM_AFECellTempUpdErr_flg : Inport
  GaISP_AFEComLost_numb : Inport  Port=2
  BMSDelay : AIWAYS_Powertrain_BMS_lib/Debounce & Delay/BMSDelay
  CFM_GaCFM_AFECellTempUpdErr_flg : AIWAYS_Powertrain_BMS_lib/Signals/OverWrite  OverWrite_Value=CaCFM_AFECellTempUpdErrOvr_flg  OverWrite_flag=CbCFM_AFECellTempUpdErrOvrSwt_flg
  Comparison4 : RelationalOperator  Operator===  OutDataTypeStr=boolean
  Constant1 : Constant  Value=CFM_RUNTIME20_MS
  Constant3 : Constant  Value=CFM_CONST0_NUMB
  Constant5 : Constant  Value=CcCFM_AFECellTempUpdErrDeb_ms
  Logical : Logic  OutDataTypeStr=boolean
  GaCFM_AFECellTempUpdErr_flg : Outport
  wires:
  CFM_GaCFM_AFECellTempUpdErr_flg/1 -> GaCFM_AFECellTempUpdErr_flg/1  "GaCFM_AFECellTempUpdErr_flg"
  BMSDelay/1 -> CFM_GaCFM_AFECellTempUpdErr_flg/1
  Constant5/1 -> BMSDelay/3
  Constant1/1 -> BMSDelay/2
  GaISP_AFEComLost_numb/1 -> Comparison4/1
  Comparison4/1 -> Logical/2
  LaCFM_AFECellTempUpdErr_flg/1 -> Logical/1
  Logical/1 -> BMSDelay/1
  Constant3/1 -> Comparison4/2

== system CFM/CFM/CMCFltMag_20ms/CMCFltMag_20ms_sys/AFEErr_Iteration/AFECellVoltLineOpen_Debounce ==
  LaCFM_AFECellVoltLineOpen_flg : Inport
  GaISP_AFEComLost_numb : Inport  Port=2
  BMSDelay : AIWAYS_Powertrain_BMS_lib/Debounce & Delay/BMSDelay
  CFM_GaCFM_AFECellVoltLineOpen_flg : AIWAYS_Powertrain_BMS_lib/Signals/OverWrite  OverWrite_Value=CaCFM_AFECellVoltLineOpenOvr_flg  OverWrite_flag=CbCFM_AFECellVoltLineOpenOvrSwt_flg
  Comparison4 : RelationalOperator  Operator===  OutDataTypeStr=boolean
  Constant1 : Constant  Value=CFM_RUNTIME20_MS
  Constant2 : Constant  Value=CFM_CONST0_NUMB
  Constant3 : Constant  Value=CcCFM_AFECellVoltLineOpenDeb_ms
  Logical : Logic  OutDataTypeStr=boolean
  GaCFM_AFECellVoltLineOpen_flg : Outport
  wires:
  LaCFM_AFECellVoltLineOpen_flg/1 -> Logical/1
  CFM_GaCFM_AFECellVoltLineOpen_flg/1 -> GaCFM_AFECellVoltLineOpen_flg/1  "GaCFM_AFECellVoltLineOpen_flg"
  BMSDelay/1 -> CFM_GaCFM_AFECellVoltLineOpen_flg/1
  Constant1/1 -> BMSDelay/2
  Constant3/1 -> BMSDelay/3
  GaISP_AFEComLost_numb/1 -> Comparison4/1
  Comparison4/1 -> Logical/2
  Logical/1 -> BMSDelay/1
  Constant2/1 -> Comparison4/2

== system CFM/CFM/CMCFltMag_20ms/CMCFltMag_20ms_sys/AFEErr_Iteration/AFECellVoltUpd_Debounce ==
  LaCFM_AFECellVoltUpdErr_flg : Inport
  GaISP_AFEComLost_numb : Inport  Port=2
  BMSDelay : AIWAYS_Powertrain_BMS_lib/Debounce & Delay/BMSDelay
  CFM_GaCFM_AFECellVoltUpdErr_flg : AIWAYS_Powertrain_BMS_lib/Signals/OverWrite  OverWrite_Value=CaCFM_AFECellVoltUpdErrOvr_flg  OverWrite_flag=CbCFM_AFECellVoltUpdErrOvrSwt_flg
  Comparison4 : RelationalOperator  Operator===  OutDataTypeStr=boolean
  Constant1 : Constant  Value=CFM_RUNTIME20_MS
  Constant3 : Constant  Value=CFM_CONST0_NUMB
  Constant5 : Constant  Value=CcCFM_AFECellVoltUpdErrDeb_ms
  Logical : Logic  OutDataTypeStr=boolean
  GaCFM_AFECellVoltUpdErr_flg : Outport
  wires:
  BMSDelay/1 -> CFM_GaCFM_AFECellVoltUpdErr_flg/1
  CFM_GaCFM_AFECellVoltUpdErr_flg/1 -> GaCFM_AFECellVoltUpdErr_flg/1  "GaCFM_AFECellVoltUpdErr_flg"
  Constant1/1 -> BMSDelay/2
  Constant5/1 -> BMSDelay/3
  Constant3/1 -> Comparison4/2
  GaISP_AFEComLost_numb/1 -> Comparison4/1
  Comparison4/1 -> Logical/2
  LaCFM_AFECellVoltUpdErr_flg/1 -> Logical/1
  Logical/1 -> BMSDelay/1

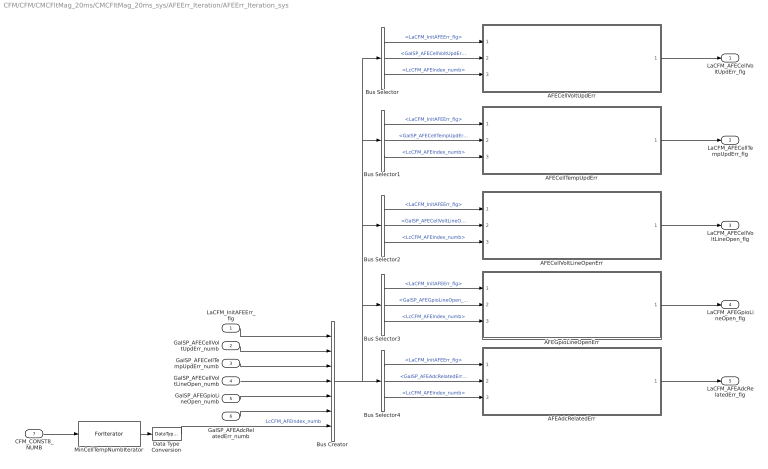
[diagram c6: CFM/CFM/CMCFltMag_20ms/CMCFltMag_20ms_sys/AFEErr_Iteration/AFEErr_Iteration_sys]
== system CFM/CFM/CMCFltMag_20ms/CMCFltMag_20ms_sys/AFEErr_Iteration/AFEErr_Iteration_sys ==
  LaCFM_InitAFEErr_flg : Inport
  GaISP_AFECellVoltUpdErr_numb : Inport  Port=2
  GaISP_AFECellTempUpdErr_numb : Inport  Port=3
  GaISP_AFECellVoltLineOpen_numb : Inport  Port=4
  GaISP_AFEGpioLineOpen_numb : Inport  Port=5
  GaISP_AFEAdcRelatedErr_numb : Inport  Port=6
  CFM_CONST8_NUMB : Inport  Port=7
  AFEAdcRelatedErr : Subsystem
  AFECellTempUpdErr : Subsystem
  AFECellVoltLineOpenErr : Subsystem
  AFECellVoltUpdErr : Subsystem
  AFEGpioLineOpenErr : Subsystem
  Bus Creator : BusCreator  Inputs=7
  Bus Selector : BusSelector  OutputSignals=LaCFM_InitAFEErr_flg,GaISP_AFECellVoltUpdErr_numb,LcCFM_AFEIndex_numb
  Bus Selector1 : BusSelector  OutputSignals=LaCFM_InitAFEErr_flg,GaISP_AFECellTempUpdErr_numb,LcCFM_AFEIndex_numb
  Bus Selector2 : BusSelector  OutputSignals=LaCFM_InitAFEErr_flg,GaISP_AFECellVoltLineOpen_numb,LcCFM_AFEIndex_numb
  Bus Selector3 : BusSelector  OutputSignals=LaCFM_InitAFEErr_flg,GaISP_AFEGpioLineOpen_numb,LcCFM_AFEIndex_numb
  Bus Selector4 : BusSelector  OutputSignals=LaCFM_InitAFEErr_flg,GaISP_AFEAdcRelatedErr_numb,LcCFM_AFEIndex_numb
  Data Type Conversion : DataTypeConversion  OutDataTypeStr=uint8
  MinCellTempNumbIterator : ForIterator  ResetStates=reset  IterationSource=external  IterationVariableDataType=int8
  LaCFM_AFECellVoltUpdErr_flg : Outport
  LaCFM_AFECellTempUpdErr_flg : Outport  Port=2
  LaCFM_AFECellVoltLineOpen_flg : Outport  Port=3
  LaCFM_AFEGpioLineOpen_flg : Outport  Port=4
  LaCFM_AFEAdcRelatedErr_flg : Outport  Port=5
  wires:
  MinCellTempNumbIterator/1 -> Data Type Conversion/1
  CFM_CONST8_NUMB/1 -> MinCellTempNumbIterator/1
  LaCFM_InitAFEErr_flg/1 -> Bus Creator/1
  GaISP_AFECellVoltUpdErr_numb/1 -> Bus Creator/2
  Data Type Conversion/1 -> Bus Creator/7  "LcCFM_AFEIndex_numb"
  Bus Creator/1 -> Bus Selector/1, Bus Selector1/1, Bus Selector2/1, Bus Selector3/1, Bus Selector4/1
  Bus Selector/1 -> AFECellVoltUpdErr/1(LaCFM_InitAFEErr_flg)  "<LaCFM_InitAFEErr_flg>"
  Bus Selector/2 -> AFECellVoltUpdErr/2(GaISP_AFECellVoltUpdErr_numb)  "<GaISP_AFECellVoltUpdErr_numb>"
  Bus Selector/3 -> AFECellVoltUpdErr/3(LcCFM_AFEIndex_numb)  "<LcCFM_AFEIndex_numb>"
  GaISP_AFECellTempUpdErr_numb/1 -> Bus Creator/3
  GaISP_AFECellVoltLineOpen_numb/1 -> Bus Creator/4
  GaISP_AFEGpioLineOpen_numb/1 -> Bus Creator/5
  GaISP_AFEAdcRelatedErr_numb/1 -> Bus Creator/6
  Bus Selector1/1 -> AFECellTempUpdErr/1(LaCFM_InitAFEErr_flg)  "<LaCFM_InitAFEErr_flg>"
  Bus Selector1/2 -> AFECellTempUpdErr/2(GaISP_AFECellTempUpdErr_numb)  "<GaISP_AFECellTempUpdErr_numb>"
  Bus Selector1/3 -> AFECellTempUpdErr/3(LcCFM_AFEIndex_numb)  "<LcCFM_AFEIndex_numb>"
  Bus Selector2/1 -> AFECellVoltLineOpenErr/1(LaCFM_InitAFEErr_flg)  "<LaCFM_InitAFEErr_flg>"
  Bus Selector2/2 -> AFECellVoltLineOpenErr/2(GaISP_AFECellVoltLineOpen_numb)  "<GaISP_AFECellVoltLineOpen_numb>"
  Bus Selector2/3 -> AFECellVoltLineOpenErr/3(LcCFM_AFEIndex_numb)  "<LcCFM_AFEIndex_numb>"
  Bus Selector3/1 -> AFEGpioLineOpenErr/1(LaCFM_InitAFEErr_flg)  "<LaCFM_InitAFEErr_flg>"
  Bus Selector3/2 -> AFEGpioLineOpenErr/2(GaISP_AFEGpioLineOpen_numb)  "<GaISP_AFEGpioLineOpen_numb>"
  Bus Selector3/3 -> AFEGpioLineOpenErr/3(LcCFM_AFEIndex_numb)  "<LcCFM_AFEIndex_numb>"
  Bus Selector4/1 -> AFEAdcRelatedErr/1(LaCFM_InitAFEErr_flg)  "<LaCFM_InitAFEErr_flg>"
  Bus Selector4/2 -> AFEAdcRelatedErr/2(GaISP_AFEAdcRelatedErr_numb)  "<GaISP_AFEAdcRelatedErr_numb>"
  Bus Selector4/3 -> AFEAdcRelatedErr/3(LcCFM_AFEIndex_numb)  "<LcCFM_AFEIndex_numb>"
  AFEGpioLineOpenErr/1(LaCFM_AFEGpioLineOpen_flg) -> LaCFM_AFEGpioLineOpen_flg/1
  AFECellVoltLineOpenErr/1(LaCFM_AFECellVoltLineOpen_flg) -> LaCFM_AFECellVoltLineOpen_flg/1
  AFECellTempUpdErr/1(LaCFM_AFECellTempUpdErr_flg) -> LaCFM_AFECellTempUpdErr_flg/1
  AFECellVoltUpdErr/1(LaCFM_AFECellVoltUpdErr_flg) -> LaCFM_AFECellVoltUpdErr_flg/1
  AFEAdcRelatedErr/1(LaCFM_AFEAdcRelatedErr_flg) -> LaCFM_AFEAdcRelatedErr_flg/1

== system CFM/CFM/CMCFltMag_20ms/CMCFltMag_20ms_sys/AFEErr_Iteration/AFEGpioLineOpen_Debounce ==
  LaCFM_AFEGpioLineOpen_flg : Inport
  GaISP_AFEComLost_numb : Inport  Port=2
  BMSDelay : AIWAYS_Powertrain_BMS_lib/Debounce & Delay/BMSDelay
  CFM_GaCFM_AFEGpioLineOpen_flg : AIWAYS_Powertrain_BMS_lib/Signals/OverWrite  OverWrite_Value=CaCFM_AFEGpioLineOpenOvr_flg  OverWrite_flag=CbCFM_AFEGpioLineOpenOvrSwt_flg
  Comparison4 : RelationalOperator  Operator===  OutDataTypeStr=boolean
  Constant1 : Constant  Value=CFM_RUNTIME20_MS
  Constant3 : Constant  Value=CFM_CONST0_NUMB
  Constant5 : Constant  Value=CcCFM_AFEGpioLineOpenDeb_ms
  Logical : Logic  OutDataTypeStr=boolean
  GaCFM_AFEGpioLineOpen_flg : Outport
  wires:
  BMSDelay/1 -> CFM_GaCFM_AFEGpioLineOpen_flg/1
  CFM_GaCFM_AFEGpioLineOpen_flg/1 -> GaCFM_AFEGpioLineOpen_flg/1  "GaCFM_AFEGpioLineOpen_flg"
  Constant1/1 -> BMSDelay/2
  Constant5/1 -> BMSDelay/3
  GaISP_AFEComLost_numb/1 -> Comparison4/1
  Comparison4/1 -> Logical/2
  LaCFM_AFEGpioLineOpen_flg/1 -> Logical/1
  Logical/1 -> BMSDelay/1
  Constant3/1 -> Comparison4/2

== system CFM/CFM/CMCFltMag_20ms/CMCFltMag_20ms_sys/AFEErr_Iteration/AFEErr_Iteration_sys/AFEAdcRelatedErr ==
  LaCFM_InitAFEErr_flg : Inport
  GaISP_AFEAdcRelatedErr_numb : Inport  Port=2
  LcCFM_AFEIndex_numb : Inport  Port=3
  AFEAdcRelatedErr_sys : Subsystem
  Assignment : Assignment  DiagnosticForDimensions=Warning  IndexOptions=Index vector (port)  Indices=1  OutputSizes=1
  Constant2 : Constant  Value=CFM_CONST14_NUMB
  LaCFM_AFEAdcRelatedErr_flg : Outport
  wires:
  LaCFM_InitAFEErr_flg/1 -> Assignment/1
  GaISP_AFEAdcRelatedErr_numb/1 -> AFEAdcRelatedErr_sys/1(GaISP_AFEAdcRelatedErr_numb)
  LcCFM_AFEIndex_numb/1 -> AFEAdcRelatedErr_sys/2(LcCFM_AFEIndex_numb), Assignment/3
  Constant2/1 -> AFEAdcRelatedErr_sys/3(CFM_CONST14_NUMB)
  AFEAdcRelatedErr_sys/1(LbCFM_AFEAdcRelatedErr_flg) -> Assignment/2
  Assignment/1 -> LaCFM_AFEAdcRelatedErr_flg/1  "LaCFM_AFEAdcRelatedErr_flg"

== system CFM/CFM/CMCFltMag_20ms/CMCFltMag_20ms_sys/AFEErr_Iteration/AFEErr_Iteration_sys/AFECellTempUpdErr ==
  LaCFM_InitAFEErr_flg : Inport
  GaISP_AFECellTempUpdErr_numb : Inport  Port=2
  LcCFM_AFEIndex_numb : Inport  Port=3
  AFECellTempUpdErr_sys : Subsystem
  Assignment : Assignment  DiagnosticForDimensions=Warning  IndexOptions=Index vector (port)  Indices=1  OutputSizes=1
  Constant2 : Constant  Value=CFM_CONST6_NUMB
  LaCFM_AFECellTempUpdErr_flg : Outport
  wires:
  Assignment/1 -> LaCFM_AFECellTempUpdErr_flg/1  "LaCFM_AFECellTempUpdErr_flg"
  AFECellTempUpdErr_sys/1(LbCFM_AFETempUpdErr_flg) -> Assignment/2
  Constant2/1 -> AFECellTempUpdErr_sys/3(CFM_CONST6_NUMB)
  LcCFM_AFEIndex_numb/1 -> Assignment/3, AFECellTempUpdErr_sys/2(LcCFM_AFEIndex_numb)
  GaISP_AFECellTempUpdErr_numb/1 -> AFECellTempUpdErr_sys/1(GaISP_AFECellTempUpdErr_numb)
  LaCFM_InitAFEErr_flg/1 -> Assignment/1

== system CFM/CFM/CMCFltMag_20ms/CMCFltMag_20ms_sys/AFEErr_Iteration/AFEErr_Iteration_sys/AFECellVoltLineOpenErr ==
  LaCFM_InitAFEErr_flg : Inport
  GaISP_AFECellVoltLineOpen_numb : Inport  Port=2
  LcCFM_AFEIndex_numb : Inport  Port=3
  AFECellVoltLineOpenErr_sys : Subsystem
  Assignment : Assignment  DiagnosticForDimensions=Warning  IndexOptions=Index vector (port)  Indices=1  OutputSizes=1
  Constant2 : Constant  Value=CFM_CONST14_NUMB
  LaCFM_AFECellVoltLineOpen_flg : Outport
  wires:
  Assignment/1 -> LaCFM_AFECellVoltLineOpen_flg/1  "LaCFM_AFECellVoltLineOpen_flg"
  AFECellVoltLineOpenErr_sys/1(LbCFM_AFECellVoltLineOpenErr_flg) -> Assignment/2
  Constant2/1 -> AFECellVoltLineOpenErr_sys/3(CFM_CONST14_NUMB)
  LcCFM_AFEIndex_numb/1 -> Assignment/3, AFECellVoltLineOpenErr_sys/2(LcCFM_AFEIndex_numb)
  GaISP_AFECellVoltLineOpen_numb/1 -> AFECellVoltLineOpenErr_sys/1(GaISP_AFECellVoltLineOpen_numb)
  LaCFM_InitAFEErr_flg/1 -> Assignment/1

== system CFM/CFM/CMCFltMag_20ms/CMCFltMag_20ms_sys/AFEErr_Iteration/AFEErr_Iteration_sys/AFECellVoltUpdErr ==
  LaCFM_InitAFEErr_flg : Inport
  GaISP_AFECellVoltUpdErr_numb : Inport  Port=2
  LcCFM_AFEIndex_numb : Inport  Port=3
  AFECellVoltUpdErr_sys : Subsystem
  Assignment : Assignment  DiagnosticForDimensions=Warning  IndexOptions=Index vector (port)  Indices=1  OutputSizes=1
  Constant2 : Constant  Value=CFM_CONST14_NUMB
  LaCFM_AFECellVoltUpdErr_flg : Outport
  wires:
  LaCFM_InitAFEErr_flg/1 -> Assignment/1
  GaISP_AFECellVoltUpdErr_numb/1 -> AFECellVoltUpdErr_sys/1(GaISP_AFECellVoltUpdErr_numb)
  LcCFM_AFEIndex_numb/1 -> AFECellVoltUpdErr_sys/2(LcCFM_AFEIndex_numb), Assignment/3
  Constant2/1 -> AFECellVoltUpdErr_sys/3(CFM_CONST14_NUMB)
  AFECellVoltUpdErr_sys/1(LbCFM_AFECellVoltUpdErr_flg) -> Assignment/2
  Assignment/1 -> LaCFM_AFECellVoltUpdErr_flg/1  "LaCFM_AFECellVoltUpdErr_flg"

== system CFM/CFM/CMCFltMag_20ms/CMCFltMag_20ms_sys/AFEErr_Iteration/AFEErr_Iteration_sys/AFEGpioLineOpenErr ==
  LaCFM_InitAFEErr_flg : Inport
  GaISP_AFEGpioLineOpen_numb : Inport  Port=2
  LcCFM_AFEIndex_numb : Inport  Port=3
  AFEGpioLineOpenErr_sys : Subsystem
  Assignment : Assignment  DiagnosticForDimensions=Warning  IndexOptions=Index vector (port)  Indices=1  OutputSizes=1
  Constant2 : Constant  Value=CFM_CONST6_NUMB
  LaCFM_AFEGpioLineOpen_flg : Outport
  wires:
  LaCFM_InitAFEErr_flg/1 -> Assignment/1
  GaISP_AFEGpioLineOpen_numb/1 -> AFEGpioLineOpenErr_sys/1(GaISP_AFEGpioLineOpen_numb)
  LcCFM_AFEIndex_numb/1 -> AFEGpioLineOpenErr_sys/2(LcCFM_AFEIndex_numb), Assignment/3
  Constant2/1 -> AFEGpioLineOpenErr_sys/3(CFM_CONST6_NUMB)
  AFEGpioLineOpenErr_sys/1(LbCFM_AFEGpioLineOpen_flg) -> Assignment/2
  Assignment/1 -> LaCFM_AFEGpioLineOpen_flg/1  "LaCFM_AFEGpioLineOpen_flg"

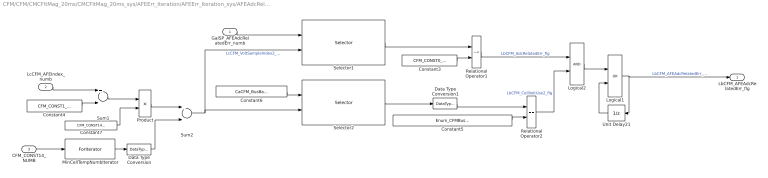
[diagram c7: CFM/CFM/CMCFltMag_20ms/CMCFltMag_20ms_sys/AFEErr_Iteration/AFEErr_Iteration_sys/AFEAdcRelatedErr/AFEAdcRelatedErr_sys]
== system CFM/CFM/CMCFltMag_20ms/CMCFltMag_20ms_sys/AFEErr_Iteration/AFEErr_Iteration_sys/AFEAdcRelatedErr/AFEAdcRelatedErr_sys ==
  GaISP_AFEAdcRelatedErr_numb : Inport
  LcCFM_AFEIndex_numb : Inport  Port=2
  CFM_CONST14_NUMB : Inport  Port=3
  Constant3 : Constant  Value=CFM_CONST0_NUMB
  Constant4 : Constant  Value=CFM_CONST1_NUMB
  Constant5 : Constant  Value=Enum_CFMBusBarCell.Enum_CFMBusBarCell_Cell
  Constant6 : Constant  Value=CaCFM_BusBarCell_enum
  Constant7 : Constant  Value=CFM_CONST14_NUMB
  Data Type Conversion : DataTypeConversion  OutDataTypeStr=uint16
  Data Type Conversion1 : DataTypeConversion
  Logical1 : Logic  Operator=OR  OutDataTypeStr=boolean
  Logical2 : Logic  OutDataTypeStr=boolean
  MinCellTempNumbIterator : ForIterator  ResetStates=reset  IterationSource=external  IterationVariableDataType=int8
  Product : Product  OutDataTypeStr=Inherit: Inherit via back propagation
  Relational Operator1 : RelationalOperator  Operator=~=  OutDataTypeStr=boolean
  Relational Operator2 : RelationalOperator  Operator===  OutDataTypeStr=boolean
  Selector1 : Selector  IndexOptions=Index vector (port)  Indices=[1 3]  OutputSizes=1
  Selector2 : Selector  IndexOptions=Index vector (port)  Indices=[1 3]  OutputSizes=1
  Sum1 : Sum  Inputs=+-  OutDataTypeStr=Inherit: Inherit via back propagation  RndMeth=Zero
  Sum2 : Sum  OutDataTypeStr=Inherit: Inherit via back propagation  RndMeth=Zero
  Unit Delay21 : UnitDelay  InitialCondition=ASWTYPE_FALSE  SampleTime=-1  StateName=StateName
  LbCFM_AFEAdcRelatedErr_flg : Outport
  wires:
  Relational Operator2/1 -> Logical2/2  "LbCFM_CellVoltUse2_flg"
  Relational Operator1/1 -> Logical2/1  "LbCFM_AdcRelatedErr_flg"
  Constant6/1 -> Selector2/1
  GaISP_AFEAdcRelatedErr_numb/1 -> Selector1/1
  Constant3/1 -> Relational Operator1/2
  Selector2/1 -> Data Type Conversion1/1
  Constant5/1 -> Relational Operator2/2
  Selector1/1 -> Relational Operator1/1
  CFM_CONST14_NUMB/1 -> MinCellTempNumbIterator/1
  MinCellTempNumbIterator/1 -> Data Type Conversion/1
  Constant4/1 -> Sum1/2
  LcCFM_AFEIndex_numb/1 -> Sum1/1
  Sum1/1 -> Product/1
  Constant7/1 -> Product/2
  Product/1 -> Sum2/1
  Data Type Conversion/1 -> Sum2/2
  Sum2/1 -> Selector1/2, Selector2/2  "LcCFM_VoltSampleIndex2_numb"
  Logical2/1 -> Logical1/1
  Unit Delay21/1 -> Logical1/2
  Logical1/1 -> LbCFM_AFEAdcRelatedErr_flg/1, Unit Delay21/1  "LbCFM_AFEAdcRelatedErr_flg"
  Data Type Conversion1/1 -> Relational Operator2/1

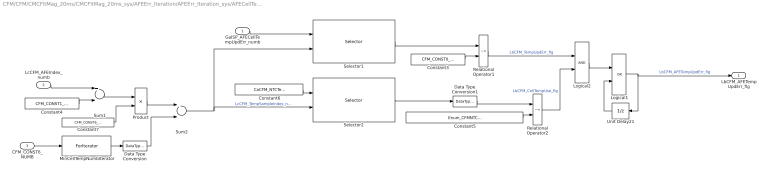
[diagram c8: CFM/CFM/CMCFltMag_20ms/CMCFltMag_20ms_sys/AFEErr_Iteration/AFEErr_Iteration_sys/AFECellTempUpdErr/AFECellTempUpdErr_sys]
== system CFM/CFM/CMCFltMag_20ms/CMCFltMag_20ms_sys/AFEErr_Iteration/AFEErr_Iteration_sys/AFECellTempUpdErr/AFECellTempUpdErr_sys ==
  GaISP_AFECellTempUpdErr_numb : Inport
  LcCFM_AFEIndex_numb : Inport  Port=2
  CFM_CONST6_NUMB : Inport  Port=3
  Constant3 : Constant  Value=CFM_CONST0_NUMB
  Constant4 : Constant  Value=CFM_CONST1_NUMB
  Constant5 : Constant  Value=Enum_CFMNTCTemp.Enum_CFMNTCTemp_NoUse
  Constant6 : Constant  Value=CaCFM_NTCTemp_enum
  Constant7 : Constant  Value=CFM_CONST6_NUMB
  Data Type Conversion : DataTypeConversion  OutDataTypeStr=uint16
  Data Type Conversion1 : DataTypeConversion
  Logical1 : Logic  Operator=OR  OutDataTypeStr=boolean
  Logical2 : Logic  OutDataTypeStr=boolean
  MinCellTempNumbIterator : ForIterator  ResetStates=reset  IterationSource=external  IterationVariableDataType=int8
  Product : Product  OutDataTypeStr=Inherit: Inherit via back propagation
  Relational Operator1 : RelationalOperator  Operator=~=  OutDataTypeStr=boolean
  Relational Operator2 : RelationalOperator  Operator=~=  OutDataTypeStr=boolean
  Selector1 : Selector  IndexOptions=Index vector (port)  Indices=[1 3]  OutputSizes=1
  Selector2 : Selector  IndexOptions=Index vector (port)  Indices=[1 3]  OutputSizes=1
  Sum1 : Sum  Inputs=+-  OutDataTypeStr=Inherit: Inherit via back propagation  RndMeth=Zero
  Sum2 : Sum  OutDataTypeStr=Inherit: Inherit via back propagation  RndMeth=Zero
  Unit Delay21 : UnitDelay  InitialCondition=ASWTYPE_FALSE  SampleTime=-1  StateName=StateName
  LbCFM_AFETempUpdErr_flg : Outport
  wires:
  Logical1/1 -> Unit Delay21/1, LbCFM_AFETempUpdErr_flg/1  "LbCFM_AFETempUpdErr_flg"
  Unit Delay21/1 -> Logical1/2
  Logical2/1 -> Logical1/1
  Sum2/1 -> Selector2/2, Selector1/2  "LcCFM_TempSampleIndex_numb"
  Data Type Conversion/1 -> Sum2/2
  Product/1 -> Sum2/1
  Constant7/1 -> Product/2
  Sum1/1 -> Product/1
  LcCFM_AFEIndex_numb/1 -> Sum1/1
  Constant4/1 -> Sum1/2
  MinCellTempNumbIterator/1 -> Data Type Conversion/1
  CFM_CONST6_NUMB/1 -> MinCellTempNumbIterator/1
  Selector1/1 -> Relational Operator1/1
  Constant5/1 -> Relational Operator2/2
  Selector2/1 -> Data Type Conversion1/1
  Constant3/1 -> Relational Operator1/2
  GaISP_AFECellTempUpdErr_numb/1 -> Selector1/1
  Constant6/1 -> Selector2/1
  Relational Operator1/1 -> Logical2/1  "LbCFM_TempUpdErr_flg"
  Relational Operator2/1 -> Logical2/2  "LbCFM_CellTempUse_flg"
  Data Type Conversion1/1 -> Relational Operator2/1

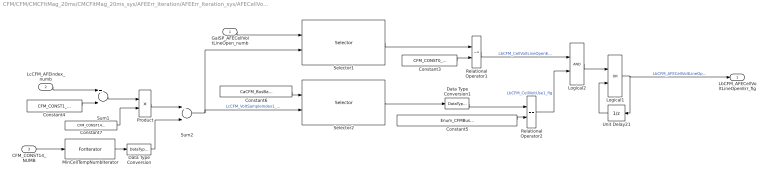
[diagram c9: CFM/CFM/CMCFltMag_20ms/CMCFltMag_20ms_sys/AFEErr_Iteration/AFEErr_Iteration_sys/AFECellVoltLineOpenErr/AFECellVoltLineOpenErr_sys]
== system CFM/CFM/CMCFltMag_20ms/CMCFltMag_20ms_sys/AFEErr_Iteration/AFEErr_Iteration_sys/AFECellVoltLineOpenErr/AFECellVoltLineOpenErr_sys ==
  GaISP_AFECellVoltLineOpen_numb : Inport
  LcCFM_AFEIndex_numb : Inport  Port=2
  CFM_CONST14_NUMB : Inport  Port=3
  Constant3 : Constant  Value=CFM_CONST0_NUMB
  Constant4 : Constant  Value=CFM_CONST1_NUMB
  Constant5 : Constant  Value=Enum_CFMBusBarCell.Enum_CFMBusBarCell_Cell
  Constant6 : Constant  Value=CaCFM_BusBarCell_enum
  Constant7 : Constant  Value=CFM_CONST14_NUMB
  Data Type Conversion : DataTypeConversion  OutDataTypeStr=uint16
  Data Type Conversion1 : DataTypeConversion
  Logical1 : Logic  Operator=OR  OutDataTypeStr=boolean
  Logical2 : Logic  OutDataTypeStr=boolean
  MinCellTempNumbIterator : ForIterator  ResetStates=reset  IterationSource=external  IterationVariableDataType=int8
  Product : Product  OutDataTypeStr=Inherit: Inherit via back propagation
  Relational Operator1 : RelationalOperator  Operator=~=  OutDataTypeStr=boolean
  Relational Operator2 : RelationalOperator  Operator===  OutDataTypeStr=boolean
  Selector1 : Selector  IndexOptions=Index vector (port)  Indices=[1 3]  OutputSizes=1
  Selector2 : Selector  IndexOptions=Index vector (port)  Indices=[1 3]  OutputSizes=1
  Sum1 : Sum  Inputs=+-  OutDataTypeStr=Inherit: Inherit via back propagation  RndMeth=Zero
  Sum2 : Sum  OutDataTypeStr=Inherit: Inherit via back propagation  RndMeth=Zero
  Unit Delay21 : UnitDelay  InitialCondition=ASWTYPE_FALSE  SampleTime=-1  StateName=StateName
  LbCFM_AFECellVoltLineOpenErr_flg : Outport
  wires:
  Logical1/1 -> Unit Delay21/1, LbCFM_AFECellVoltLineOpenErr_flg/1  "LbCFM_AFECellVoltLineOpenErr_flg"
  Unit Delay21/1 -> Logical1/2
  Logical2/1 -> Logical1/1
  Sum2/1 -> Selector2/2, Selector1/2  "LcCFM_VoltSampleIndex1_numb"
  Data Type Conversion/1 -> Sum2/2
  Product/1 -> Sum2/1
  Constant7/1 -> Product/2
  Sum1/1 -> Product/1
  LcCFM_AFEIndex_numb/1 -> Sum1/1
  Constant4/1 -> Sum1/2
  MinCellTempNumbIterator/1 -> Data Type Conversion/1
  CFM_CONST14_NUMB/1 -> MinCellTempNumbIterator/1
  Selector1/1 -> Relational Operator1/1
  Constant5/1 -> Relational Operator2/2
  Selector2/1 -> Data Type Conversion1/1
  Constant3/1 -> Relational Operator1/2
  GaISP_AFECellVoltLineOpen_numb/1 -> Selector1/1
  Constant6/1 -> Selector2/1
  Relational Operator1/1 -> Logical2/1  "LbCFM_CellVoltLineOpenErr_flg"
  Relational Operator2/1 -> Logical2/2  "LbCFM_CellVoltUse1_flg"
  Data Type Conversion1/1 -> Relational Operator2/1

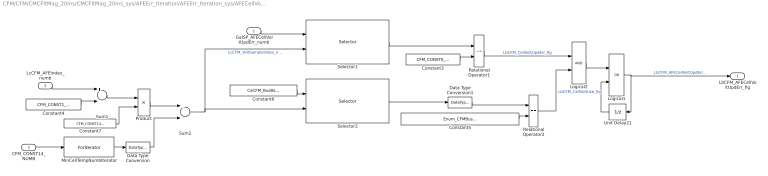
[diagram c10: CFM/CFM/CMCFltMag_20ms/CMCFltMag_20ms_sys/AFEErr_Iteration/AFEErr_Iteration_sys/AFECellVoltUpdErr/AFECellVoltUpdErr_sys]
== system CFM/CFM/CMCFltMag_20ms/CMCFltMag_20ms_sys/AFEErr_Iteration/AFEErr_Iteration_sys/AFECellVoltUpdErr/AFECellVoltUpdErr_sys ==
  GaISP_AFECellVoltUpdErr_numb : Inport
  LcCFM_AFEIndex_numb : Inport  Port=2
  CFM_CONST14_NUMB : Inport  Port=3
  Constant3 : Constant  Value=CFM_CONST0_NUMB
  Constant4 : Constant  Value=CFM_CONST1_NUMB
  Constant5 : Constant  Value=Enum_CFMBusBarCell.Enum_CFMBusBarCell_Cell
  Constant6 : Constant  Value=CaCFM_BusBarCell_enum
  Constant7 : Constant  Value=CFM_CONST14_NUMB
  Data Type Conversion : DataTypeConversion  OutDataTypeStr=uint16
  Data Type Conversion1 : DataTypeConversion
  Logical1 : Logic  Operator=OR  OutDataTypeStr=boolean
  Logical2 : Logic  OutDataTypeStr=boolean
  MinCellTempNumbIterator : ForIterator  ResetStates=reset  IterationSource=external  IterationVariableDataType=int8
  Product : Product  OutDataTypeStr=Inherit: Inherit via back propagation
  Relational Operator1 : RelationalOperator  Operator=~=  OutDataTypeStr=boolean
  Relational Operator2 : RelationalOperator  Operator===  OutDataTypeStr=boolean
  Selector1 : Selector  IndexOptions=Index vector (port)  Indices=[1 3]  OutputSizes=1
  Selector2 : Selector  IndexOptions=Index vector (port)  Indices=[1 3]  OutputSizes=1
  Sum1 : Sum  Inputs=+-  OutDataTypeStr=Inherit: Inherit via back propagation  RndMeth=Zero
  Sum2 : Sum  OutDataTypeStr=Inherit: Inherit via back propagation  RndMeth=Zero
  Unit Delay21 : UnitDelay  InitialCondition=ASWTYPE_FALSE  SampleTime=-1  StateName=StateName
  LbCFM_AFECellVoltUpdErr_flg : Outport
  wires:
  Relational Operator2/1 -> Logical2/2  "LbCFM_CellVoltUse_flg"
  Relational Operator1/1 -> Logical2/1  "LbCFM_CellVoltUpdErr_flg"
  Constant6/1 -> Selector2/1
  GaISP_AFECellVoltUpdErr_numb/1 -> Selector1/1
  Constant3/1 -> Relational Operator1/2
  Selector2/1 -> Data Type Conversion1/1
  Constant5/1 -> Relational Operator2/2
  Selector1/1 -> Relational Operator1/1
  CFM_CONST14_NUMB/1 -> MinCellTempNumbIterator/1
  MinCellTempNumbIterator/1 -> Data Type Conversion/1
  Constant4/1 -> Sum1/2
  LcCFM_AFEIndex_numb/1 -> Sum1/1
  Sum1/1 -> Product/1
  Constant7/1 -> Product/2
  Product/1 -> Sum2/1
  Data Type Conversion/1 -> Sum2/2
  Sum2/1 -> Selector1/2, Selector2/2  "LcCFM_VoltSampleIndex_numb"
  Logical2/1 -> Logical1/1
  Unit Delay21/1 -> Logical1/2
  Logical1/1 -> LbCFM_AFECellVoltUpdErr_flg/1, Unit Delay21/1  "LbCFM_AFECellVoltUpdErr_flg"
  Data Type Conversion1/1 -> Relational Operator2/1

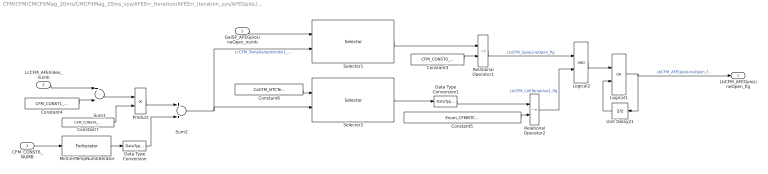
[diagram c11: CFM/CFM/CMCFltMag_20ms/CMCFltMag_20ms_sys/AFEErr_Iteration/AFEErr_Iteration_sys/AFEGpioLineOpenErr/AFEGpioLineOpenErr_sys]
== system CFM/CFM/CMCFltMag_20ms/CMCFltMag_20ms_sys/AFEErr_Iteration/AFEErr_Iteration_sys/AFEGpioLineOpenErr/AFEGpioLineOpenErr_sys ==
  GaISP_AFEGpioLineOpen_numb : Inport
  LcCFM_AFEIndex_numb : Inport  Port=2
  CFM_CONST6_NUMB : Inport  Port=3
  Constant3 : Constant  Value=CFM_CONST0_NUMB
  Constant4 : Constant  Value=CFM_CONST1_NUMB
  Constant5 : Constant  Value=Enum_CFMNTCTemp.Enum_CFMNTCTemp_NoUse
  Constant6 : Constant  Value=CaCFM_NTCTemp_enum
  Constant7 : Constant  Value=CFM_CONST6_NUMB
  Data Type Conversion : DataTypeConversion  OutDataTypeStr=uint16
  Data Type Conversion1 : DataTypeConversion
  Logical1 : Logic  Operator=OR  OutDataTypeStr=boolean
  Logical2 : Logic  OutDataTypeStr=boolean
  MinCellTempNumbIterator : ForIterator  ResetStates=reset  IterationSource=external  IterationVariableDataType=int8
  Product : Product  OutDataTypeStr=Inherit: Inherit via back propagation
  Relational Operator1 : RelationalOperator  Operator=~=  OutDataTypeStr=boolean
  Relational Operator2 : RelationalOperator  Operator=~=  OutDataTypeStr=boolean
  Selector1 : Selector  IndexOptions=Index vector (port)  Indices=[1 3]  OutputSizes=1
  Selector2 : Selector  IndexOptions=Index vector (port)  Indices=[1 3]  OutputSizes=1
  Sum1 : Sum  Inputs=+-  OutDataTypeStr=Inherit: Inherit via back propagation  RndMeth=Zero
  Sum2 : Sum  OutDataTypeStr=Inherit: Inherit via back propagation  RndMeth=Zero
  Unit Delay21 : UnitDelay  InitialCondition=ASWTYPE_FALSE  SampleTime=-1  StateName=StateName
  LbCFM_AFEGpioLineOpen_flg : Outport
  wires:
  Relational Operator2/1 -> Logical2/2  "LbCFM_CellTempUse1_flg"
  Relational Operator1/1 -> Logical2/1  "LbCFM_GpioLineOpen_flg"
  Constant6/1 -> Selector2/1
  GaISP_AFEGpioLineOpen_numb/1 -> Selector1/1
  Constant3/1 -> Relational Operator1/2
  Selector2/1 -> Data Type Conversion1/1
  Constant5/1 -> Relational Operator2/2
  Selector1/1 -> Relational Operator1/1
  CFM_CONST6_NUMB/1 -> MinCellTempNumbIterator/1
  MinCellTempNumbIterator/1 -> Data Type Conversion/1
  Constant4/1 -> Sum1/2
  LcCFM_AFEIndex_numb/1 -> Sum1/1
  Sum1/1 -> Product/1
  Constant7/1 -> Product/2
  Product/1 -> Sum2/1
  Data Type Conversion/1 -> Sum2/2
  Sum2/1 -> Selector1/2, Selector2/2  "LcCFM_TempSampleIndex1_numb"
  Logical2/1 -> Logical1/1
  Unit Delay21/1 -> Logical1/2
  Logical1/1 -> LbCFM_AFEGpioLineOpen_flg/1, Unit Delay21/1  "LbCFM_AFEGpioLineOpen_flg"
  Data Type Conversion1/1 -> Relational Operator2/1
